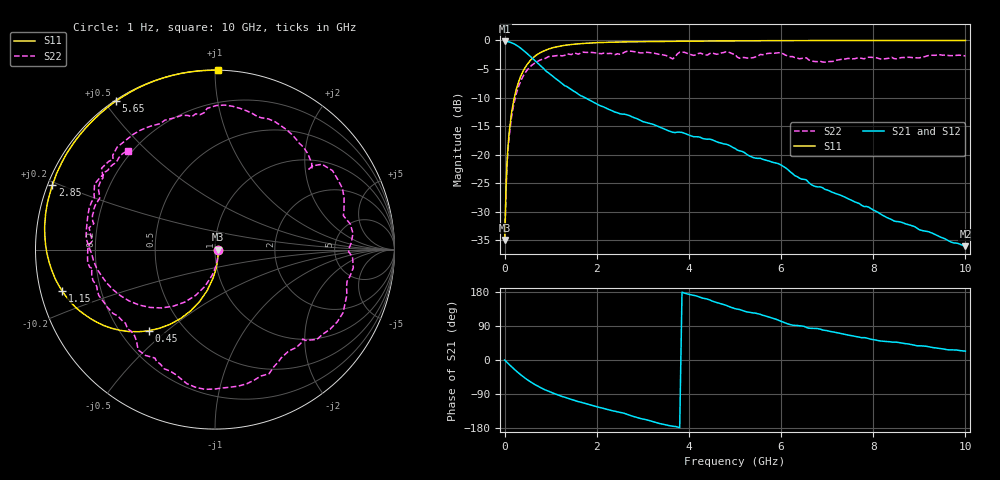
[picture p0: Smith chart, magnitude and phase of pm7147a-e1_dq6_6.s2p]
# GHz S DB R 50
! S-Parameters data
! Freq  dbS11  angS11  dbS21  angS21  dbS12  angS12  dbS22  angS22
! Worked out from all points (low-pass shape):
!   279 points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, 1 Hz to 10 GHz, reference 50 ohm
!   highest |S21| = -0.16 dB at 19.95 kHz (marker M1); lowest = -36.1 dB at 10 GHz (marker M2)
!   |S21| within 3 dB of the highest: start of sweep to 605.9 MHz
!   lowest |S11| = -35.0 dB at 15.85 kHz (marker M3), VSWR 1.04, Z = 51.8 - j0.00257 ohm
!   |S11| at or under -10 dB: start of sweep to 211.9 MHz
!   |S22| runs from -35.0 to -1.9 dB; largest |S21 - S12| = 0
!   S11 on the Smith chart (normalised r, x): 1 Hz: 1.04, -0.00; 450 MHz: 0.32, -0.44; 1.15 GHz: 0.06, -0.13; 2.85 GHz: 0.01, +0.19; 5.65 GHz: 0.00, +0.54; 10 GHz: 0.00, +1.02
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1e-09  -34.97 -0.0  -0.16 -0.0  -0.16 -0.0  -34.97 -0.0
1.58489e-05  -34.97 -0.1  -0.16 -0.0  -0.16 -0.0  -34.97 -0.1
1.99526e-05  -34.97 -0.1  -0.16 -0.0  -0.16 -0.0  -34.97 -0.1
0.05011872  -21.86 -82.1  -0.19 -6.0  -0.19 -6.0  -22.52 -82.8
0.15  -12.73 -100.7  -0.40 -17.6  -0.40 -17.6  -13.43 -105.4
0.45  -4.68 -129.2  -2.02 -48.4  -2.02 -48.4  -5.62 -143.9
0.75  -2.26 -148.3  -4.21 -70.8  -4.21 -70.8  -3.52 -170.9
1.15  -1.08 -165.0  -6.93 -92.0  -6.93 -92.0  -2.64 161.9
1.7  -0.53 179.6  -9.84 -113.0  -9.84 -113.0  -2.05 133.7
2.3  -0.31 167.4  -12.20 -132.6  -12.20 -132.6  -2.26 103.9
2.85  -0.22 158.3  -13.64 -150.7  -13.64 -150.7  -2.01 77.3
3.35  -0.16 150.9  -15.14 -167.3  -15.14 -167.3  -2.43 51.5
3.75  -0.13 145.5  -16.06 -176.7  -16.06 -176.7  -2.35 38.6
4.25  -0.11 139.2  -16.98 165.1  -16.98 165.1  -2.23 6.7
4.8  -0.08 132.8  -18.16 144.6  -18.16 144.6  -1.99 -26.3
5.05  -0.07 130.0  -19.20 134.2  -19.20 134.2  -2.93 -45.2
5.65  -0.05 123.7  -20.93 116.7  -20.93 116.7  -2.40 -73.1
6.1  -0.04 119.3  -22.34 97.5  -22.34 97.5  -2.59 -105.2
6.7  -0.02 113.7  -25.46 83.4  -25.46 83.4  -3.66 -133.2
7.65  -0.01 105.6  -28.44 61.8  -28.44 61.8  -3.08 -165.8
8.35  -0.01 100.2  -31.23 48.3  -31.23 48.3  -3.10 172.7
10  -0.00 89.1  -36.05 23.3  -36.05 23.3  -2.72 131.6
